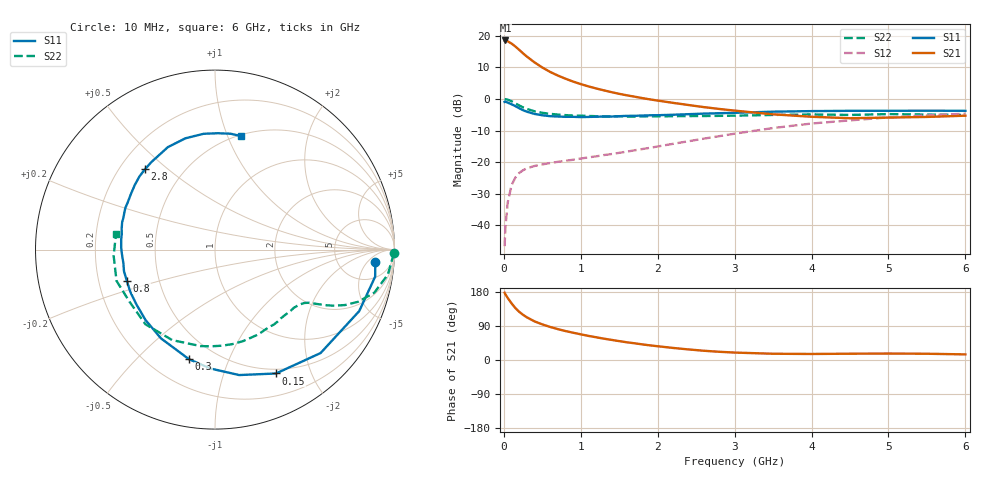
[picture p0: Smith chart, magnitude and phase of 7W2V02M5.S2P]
! Infineon Technologies  Discrete & RF Semiconductors
! BFS17W
! Si NPN RF Bipolar Junction Transistor in SOT323
! VCE = 2 V  IC = 2.5 mA
! Common Emitter S-Parameters:  August  1999
# GHz  S  MA  R  50
!  f  S11  S21  S12  S22
! GHz  MAG  ANG  MAG  ANG  MAG  ANG  MAG  ANG
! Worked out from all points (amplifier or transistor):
!   36 points, 10 MHz to 6 GHz, reference 50 ohm
!   highest |S21| = 18.5 dB at 20 MHz (marker M1)
!   |S21| within 3 dB of that: start of sweep to 201.2 MHz
!   unconditionally stable (mu >= 1): 737.4 MHz to end of sweep
!   at 250 MHz: K = 0.41, MSG = 18.5 dB, |S12| = -22.5 dB
!   at 1.4 GHz: K = 1.33, MAG = 6.3 dB, |S12| = -17.4 dB
!   at 6 GHz: K = 1.11, MAG = -2.3 dB, |S12| = -4.7 dB
!   S11 on the Smith chart (normalised r, x): 10 MHz: 12, -9; 150 MHz: 0.45, -1.51; 300 MHz: 0.36, -0.72; 800 MHz: 0.32, -0.15; 2.8 GHz: 0.30, +0.42; 6 GHz: 0.51, +1.12
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0.01  0.896 -4.6  8.372 177.4  0.0047 82.3  0.9975 -1.2
0.02  0.905 -9.6  8.397 173.5  0.0091 82.4  0.9878 -3.3
0.05  0.8735 -23.1  8.15 163.8  0.023 77.1  0.9733 -8.2
0.1  0.8236 -44.4  7.508 149.6  0.0432 67.3  0.9197 -15.1
0.15  0.7693 -63.8  6.733 137.0  0.0572 57.4  0.8495 -20.0
0.2  0.7118 -79.1  5.963 127.1  0.0675 52.0  0.7873 -23.1
0.25  0.663 -92.2  5.248 119.2  0.0746 47.2  0.7343 -25.2
0.3  0.6274 -103.4  4.666 112.5  0.08 44.3  0.6953 -26.5
0.4  0.579 -121.3  3.77 101.8  0.0872 40.9  0.6369 -28.3
0.5  0.5512 -134.6  3.14 94.0  0.0921 39.8  0.6032 -29.4
0.6  0.5338 -145.1  2.677 87.3  0.0968 39.7  0.5805 -30.8
0.8  0.521 -160.7  2.09 76.5  0.1053 41.5  0.5545 -34.5
0.9  0.5212 -166.7  1.88 72.0  0.1091 43.0  0.5459 -36.4
1.1  0.5191 -177.2  1.578 63.6  0.1191 45.9  0.5375 -41.0
1.3  0.5257 174.0  1.366 56.3  0.1294 48.8  0.5303 -46.4
1.6  0.5395 163.5  1.139 46.7  0.1469 52.7  0.5268 -54.7
2.2  0.5619 146.4  0.866 31.8  0.1951 58.3  0.5332 -73.0
2.8  0.594 131.0  0.694 21.7  0.2576 59.3  0.5394 -92.5
3.5  0.6284 114.7  0.571 16.5  0.3463 55.4  0.5578 -115.3
4.5  0.6484 95.6  0.495 16.6  0.4576 43.8  0.5579 -148.7
5.5  0.6515 82.2  0.519 16.5  0.5482 31.8  0.5657 -176.6
6  0.6486 77.1  0.543 14.8  0.5841 26.1  0.5584 171.2
